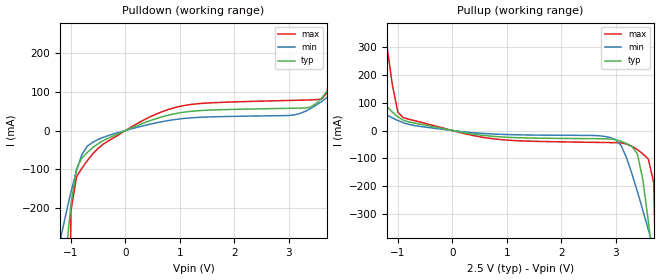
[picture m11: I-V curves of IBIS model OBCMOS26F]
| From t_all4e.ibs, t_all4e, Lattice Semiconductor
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|   OBCMOS26F
[Model]   OBCMOS26F
Model_type   Output
Polarity   Non-Inverting
C_comp   2pF   2pF   2pF
[Temperature Range]   25.0000   125.0000   -40.0000
[Voltage Range]   2.5000V   2.3000V   2.7000V
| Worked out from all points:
|   slope of the pulldown table from 0 to 0.375 V, typ, clamps not added: 17.5 ohm
|   slope of the pullup table from 0 to 0.375 V, typ, clamps not added: 28.8 ohm
[Pulldown]
|voltage   I(typ)   I(min)   I(max)
-2.5V     -2.905A    -1.222A    -25.79A
-1.2V     -491mA     -283.3mA   -2.511A
-1.1V     -328.4mA   -217.8mA   -1.031A
-900mV    -97.98mA   -102.8mA   -118.9mA
-700mV    -56.12mA   -39.95mA   -77.2mA
-500mV    -33.39mA   -22.91mA   -45.31mA
1V        45.55mA    29.8mA     62.07mA
3.2V      57.54mA    43.52mA    77.91mA
3.7V      100.3mA    84.65mA    95.81mA
3.9V      142.8mA    108.8mA    325.2mA
4.4V      272.4mA    183.3mA    1.132A
5V        456.4mA    288.4mA    2.175A
[Pullup]
|voltage   I(typ)   I(min)   I(max)
-2.5V     447.3mA    250.8mA    2.513A
-2.2V     355mA      198.3mA    1.983A
-1.3V     109.3mA    66.63mA    457.2mA
-1V       49.14mA    36.01mA    65.78mA
-900mV    37.02mA    28.1mA     46.41mA
2.9V      -30.64mA   -25.34mA   -43.53mA
3.1V      -38.99mA   -53.94mA   -44.81mA
3.4V      -84.17mA   -221mA     -69.05mA
3.6V      -327mA     -357.4mA   -102.9mA
3.7V      -494.9mA   -427.7mA   -189.3mA
3.8V      -670.7mA   -498.8mA   -1.025A
5V        -2.912A    -1.377A    -22.13A
[Ramp]
| variable   typ   min   max
dV/dt_r   0.7745/0.3336ns   0.4842/0.5245ns   1.0778/0.2014ns
dV/dt_f   1.0879/0.5965ns   0.8580/1.2567ns   1.2705/0.2905ns
